(* Logix 5000 AddOnInstructionDefinition export AMCI_ANG1E_Run_Blend_Move; software revision 20.03 *)

ADD_ON_INSTRUCTION AMCI_ANG1E_Run_Blend_Move   (* revision 5.0, vendor AMCI, ExecuteEnableInFalse *)
// Revision note:
// Version 5.0 added the (hidden) ability to program the motor current and unlatched the error bit if the rung goes false.
VAR_INPUT
   Axis_Status_bits : INT; {required}
   slot_axis_number : INT; {required}
   Direction_0_for_CW_1_for_CCW : BOOL; {required}
   Type_0_for_standard_1_for_indexed : BOOL;
   motor_current : INT;
END_VAR
VAR_IN_OUT
   AMCI_ANG1E_output_data : INT[10]; {required}
END_VAR
VAR_OUTPUT
   EN : BOOL; {access Read Only, visible}
   ER : BOOL; {access Read Only, visible}
END_VAR
VAR
   command_data_block : INT[10];
        [0]   // Command Bits MSW
        [1]   // Command Bits LSW
        [2]   // Upper Target Position
        [3]   // Lower Target Position
        [4]   // Upper Programmed Speed
        [5]   // Lower Programmed Speed
   index : INT;
END_VAR

ROUTINE EnableInFalse   (* ladder *)
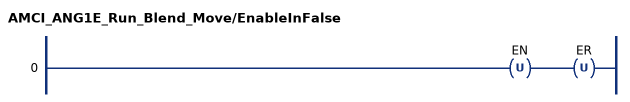
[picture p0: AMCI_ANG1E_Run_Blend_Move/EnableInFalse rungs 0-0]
   0: OTU(EN)OTU(ER);
END_ROUTINE

ROUTINE Logic   (* ladder *)
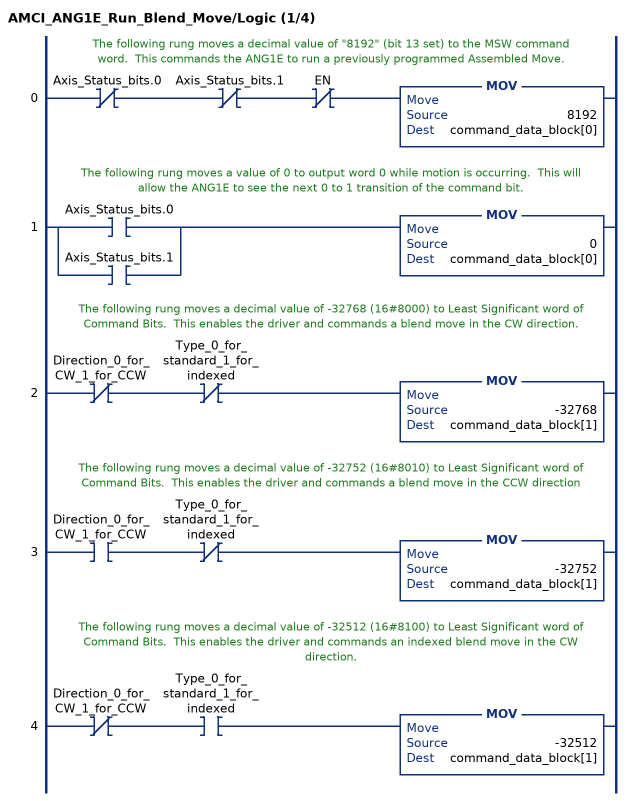
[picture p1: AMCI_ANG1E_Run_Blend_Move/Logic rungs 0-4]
   // The following rung moves a decimal value of "8192" (bit 13 set) to the MSW command word.  This commands the ANG1E to run a previously programmed Assembled Move.
   0: XIO(Axis_Status_bits.0)XIO(Axis_Status_bits.1)XIO(EN)MOV(8192,command_data_block[0]);
   // The following rung moves a value of 0 to output word 0 while motion is occurring.  This will allow the ANG1E to see the next 0 to 1 transition of the command bit.
   1: [XIC(Axis_Status_bits.0) ,XIC(Axis_Status_bits.1) ]MOV(0,command_data_block[0]);
   // The following rung moves a decimal value of -32768 (16#8000) to Least Significant word of Command Bits.  This enables the driver and commands a blend move in the CW direction.
   2: XIO(Direction_0_for_CW_1_for_CCW)XIO(Type_0_for_standard_1_for_indexed)MOV(-32768,command_data_block[1]);
   // The following rung moves a decimal value of -32752 (16#8010) to Least Significant word of Command Bits.  This enables the driver and commands a blend move in the CCW direction
   3: XIC(Direction_0_for_CW_1_for_CCW)XIO(Type_0_for_standard_1_for_indexed)MOV(-32752,command_data_block[1]);
   // The following rung moves a decimal value of -32512 (16#8100) to Least Significant word of Command Bits.  This enables the driver and commands an indexed blend move in the CW direction.
   4: XIO(Direction_0_for_CW_1_for_CCW)XIC(Type_0_for_standard_1_for_indexed)MOV(-32512,command_data_block[1]);
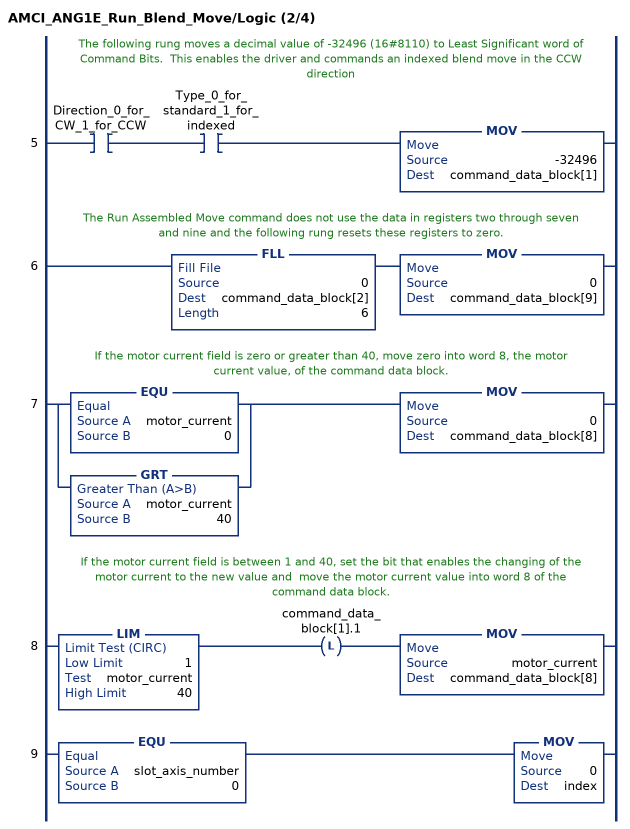
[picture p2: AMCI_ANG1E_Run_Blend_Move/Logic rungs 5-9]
   // The following rung moves a decimal value of -32496 (16#8110) to Least Significant word of Command Bits.  This enables the driver and commands an indexed blend move in the CCW direction
   5: XIC(Direction_0_for_CW_1_for_CCW)XIC(Type_0_for_standard_1_for_indexed)MOV(-32496,command_data_block[1]);
   // The Run Assembled Move command does not use the data in registers two through seven and nine and the following rung resets these registers to zero.
   6: FLL(0,command_data_block[2],6)MOV(0,command_data_block[9]);
   // If the motor current field is zero or greater than 40, move zero into word 8, the motor current value, of the command data block.
   7: [EQU(motor_current,0) ,GRT(motor_current,40) ]MOV(0,command_data_block[8]);
   // If the motor current field is between 1 and 40, set the bit that enables the changing of the motor current to the new value and  move the motor current value into word 8 of the command data block.
   8: LIM(1,motor_current,40)OTL(command_data_block[1].1)MOV(motor_current,command_data_block[8]);
   9: EQU(slot_axis_number,0)MOV(0,index);
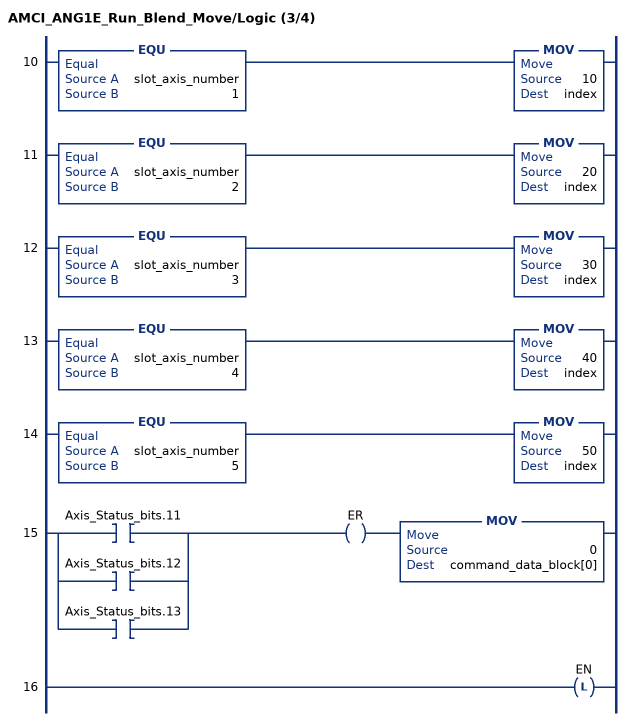
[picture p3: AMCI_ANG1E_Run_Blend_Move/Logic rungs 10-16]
   10: EQU(slot_axis_number,1)MOV(10,index);
   11: EQU(slot_axis_number,2)MOV(20,index);
   12: EQU(slot_axis_number,3)MOV(30,index);
   13: EQU(slot_axis_number,4)MOV(40,index);
   14: EQU(slot_axis_number,5)MOV(50,index);
   15: [XIC(Axis_Status_bits.11) ,XIC(Axis_Status_bits.12) ,XIC(Axis_Status_bits.13) ]OTE(ER)MOV(0,command_data_block[0]);
   16: OTL(EN);
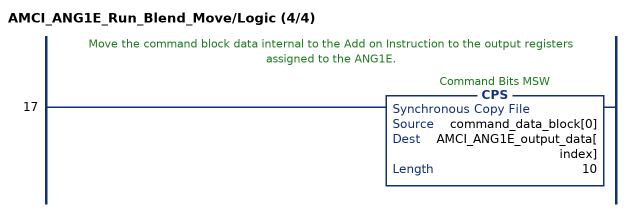
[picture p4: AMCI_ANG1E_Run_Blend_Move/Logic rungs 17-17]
   // Move the command block data internal to the Add on Instruction to the output registers assigned to the ANG1E.
   17: CPS(command_data_block[0],AMCI_ANG1E_output_data[index],10);
END_ROUTINE
END_ADD_ON_INSTRUCTION
